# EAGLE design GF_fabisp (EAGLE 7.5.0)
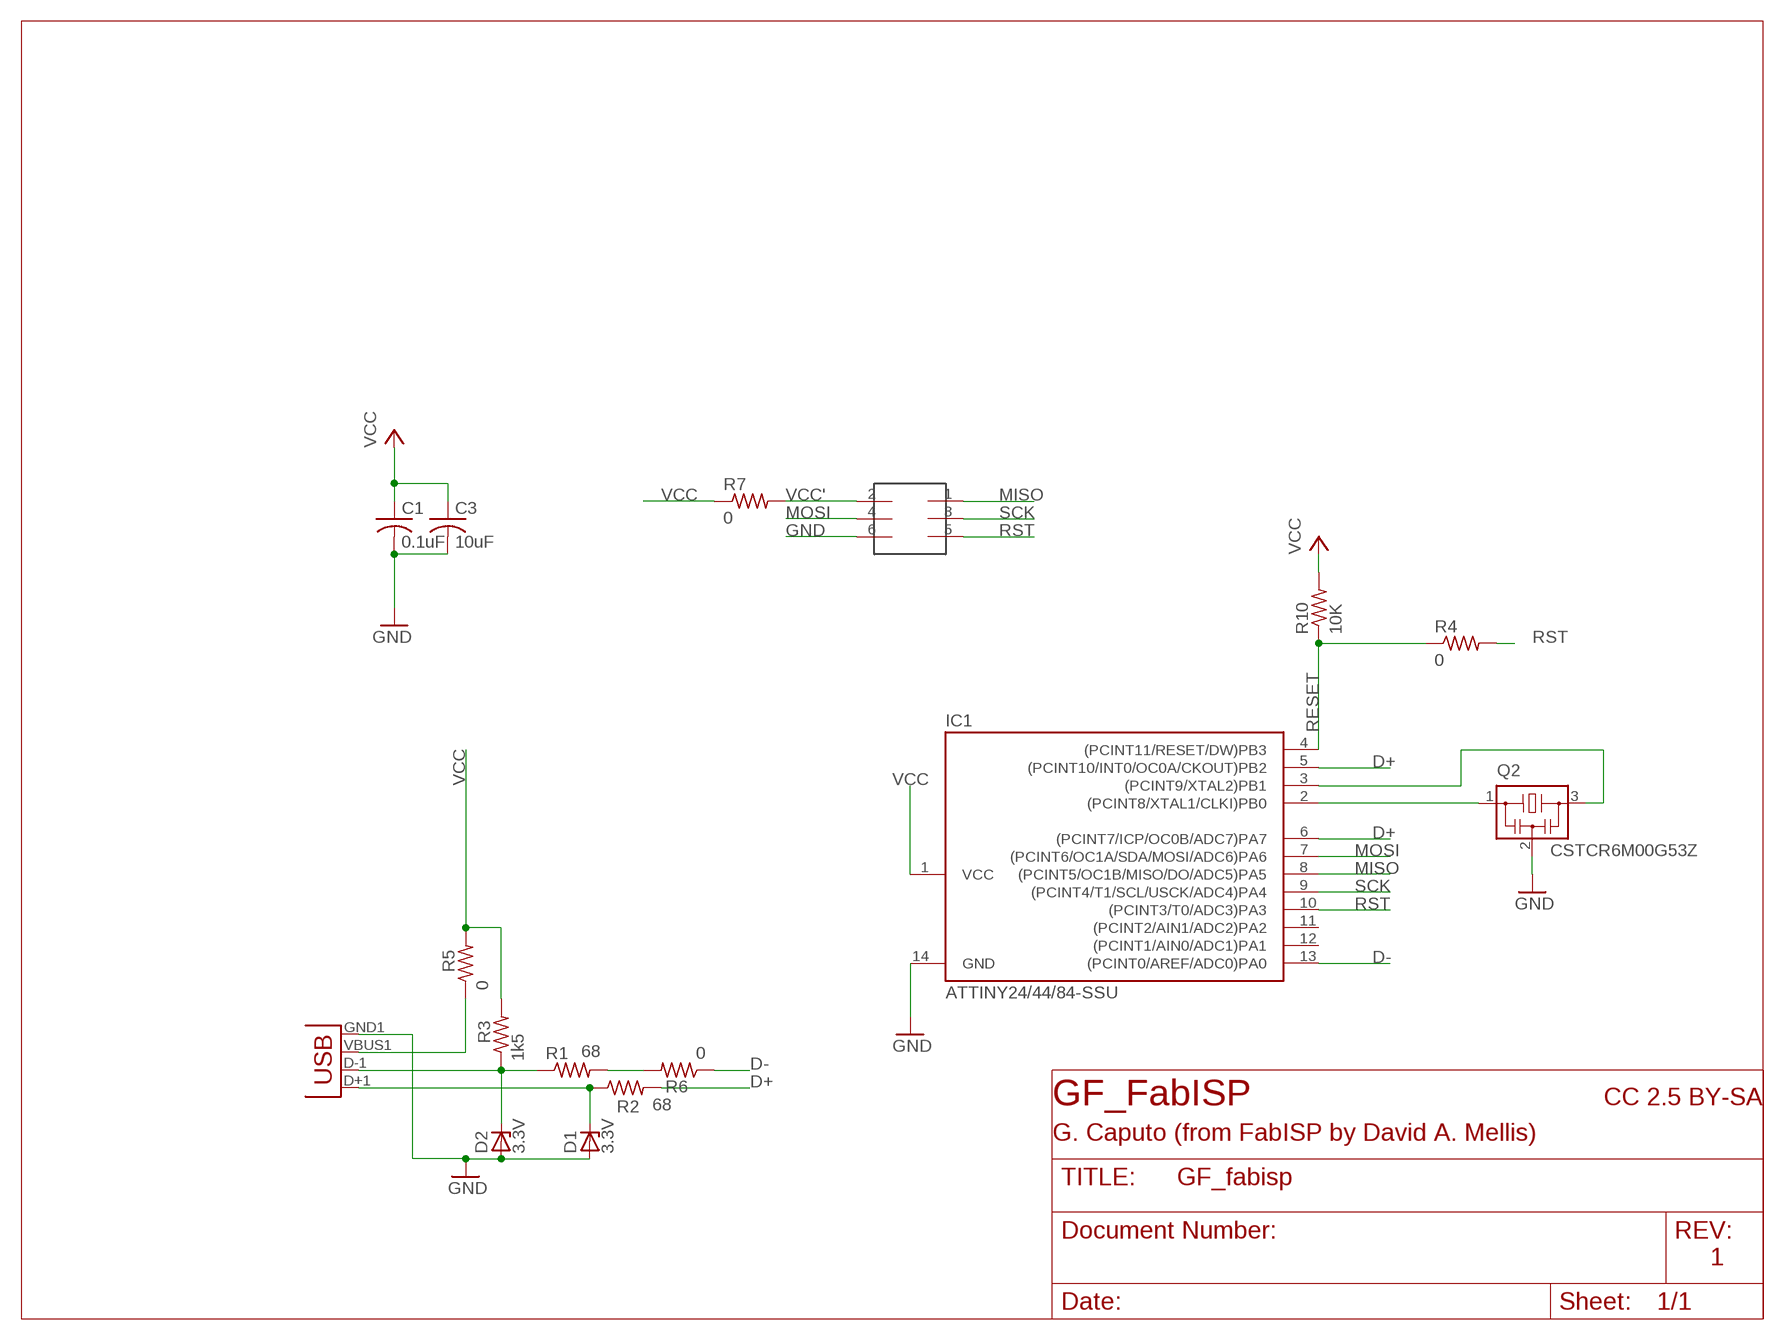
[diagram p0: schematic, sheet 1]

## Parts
C1  0.1uF  C-USC1206  [C1206]
C3  10uF  C-USC1206  [C1206]
D1  3.3V  ZENER_DIODESOD123  [SOD123]
D2  3.3V  ZENER_DIODESOD123  [SOD123]
IC1  ATTINY24/44/84-SSU  [SOIC14]
JP1  USBA-SMD-MALE  [USB-A-SMT-MALE]
Q2  CSTCR6M00G53Z  [CSTCR6M]
R1  68  R-US_R1206  [R1206]
R2  68  R-US_R1206  [R1206]
R3  1k5  R-US_R1206  [R1206]
R4  0  R-US_R1206  [R1206]
R5  0  R-US_R1206  [R1206]
R6  0  R-US_R1206  [R1206]
R7  0  R-US_R1206  [R1206]
R10  10K  R-US_R1206  [R1206]
U$1  2X3HEADER  [2X3_SMD]

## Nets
D+: IC1.5((PCINT10/INT0/OC0A/CKOUT)PB2) IC1.6((PCINT7/ICP/OC0B/ADC7)PA7) R2.2
D-: IC1.13((PCINT0/AREF/ADC0)PA0) R6.1
GND: C1.2 C3.2 D1.ANODE D2.ANODE IC1.14(GND) JP1.GND1(GND) Q2.2 U$1.6
MISO: IC1.8((PCINT5/OC1B/MISO/DO/ADC5)PA5) U$1.1
MOSI: IC1.7((PCINT6/OC1A/SDA/MOSI/ADC6)PA6) U$1.4
N$1: D2.CATHODE JP1.D-1(D-) R1.1 R3.1
N$2: D1.CATHODE JP1.D+1(D+) R2.1
N$4: IC1.2((PCINT8/XTAL1/CLKI)PB0) Q2.1
N$5: IC1.3((PCINT9/XTAL2)PB1) Q2.3
N$6: JP1.VBUS1(VBUS) R5.1
N$7: R1.2 R6.2
RESET: IC1.4((PCINT11/RESET/DW)PB3) R4.1 R10.1
RST: IC1.10((PCINT3/T0/ADC3)PA3) R4.2 U$1.5
SCK: IC1.9((PCINT4/T1/SCL/USCK/ADC4)PA4) U$1.3
VCC: C1.1 C3.1 IC1.1(VCC) R3.2 R5.2 R7.1 R10.2
VCC': R7.2 U$1.2
Unconnected: IC1.11((PCINT2/AIN1/ADC2)PA2) IC1.12((PCINT1/AIN0/ADC1)PA1)

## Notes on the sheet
- GF_FabISP | CC 2.5 BY-SA
- G. Caputo (from FabISP by David A. Mellis)
- 1

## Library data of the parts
C1 = rcl-ez:C-US: CAPACITOR, American symbol
C3 = rcl:C-US: CAPACITOR, American symbol
D1 D2 = ng:ZENER_DIODE: zener diode
IC1 = attiny24_44_84:ATTINY24/44/84
JP1 = SparkFun-Connectors:USB: USB Connectors USB-B-PTH is fully proven SKU : PRT-00139/CONN-08278 USB-miniB is fully proven SKU : PRT-00587 USB-A-PCB is untested. USB-A-H is throughly reviewed, but untested. Spark Fun Electronics SKU : PRT-00437 USB-B-SMT is throughly reviewed, but untested. Needs silkscreen touching up.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
Q2 = FablabTorino:CSTCR: Resonator Source: murata.co.jp; MPN: CSTCR6M00G53-R0; OC_FARNELL: 1170434; OC_NEWARK: 25M8759
R1-R3 R5 R6 R10 = rcl-ez:R-US_: RESISTOR, American symbol
R4 R7 = rcl:R-US_: RESISTOR, American symbol
U$1 = mellis:2X3HEADER

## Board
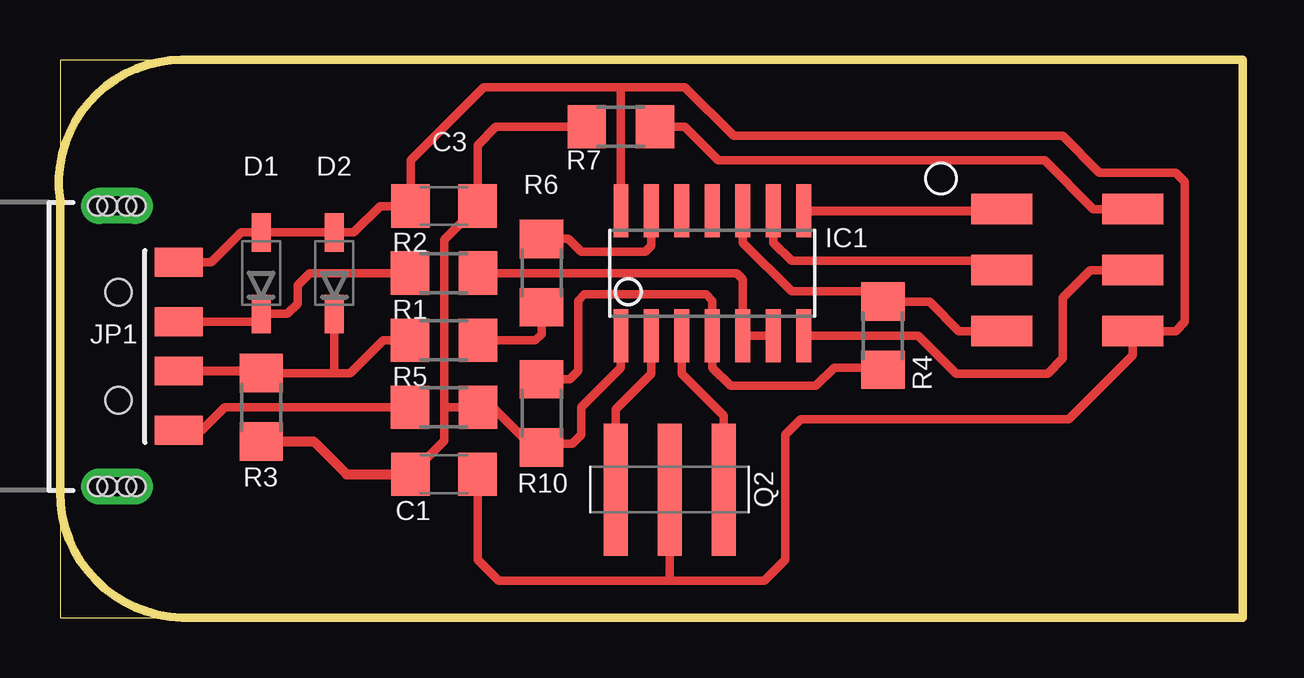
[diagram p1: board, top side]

Size 49.33 x 23.23 mm. Coordinates in mm from the lower left corner, seen from the top.
Outline: 0,0 49.33,0 49.33,23.23 0,23.23 0,0
Copper layers (1*16): Top 0.035mm / dielectric 1.5mm / Bottom 0.035mm
Design rules "default": minimum track width 10mil, minimum drill 24mil, track to track 8mil, track to pad 8mil, pad to pad 8mil, via to via 8mil, smd to smd 8mil, copper to edge 40mil, drill to drill 8mil, minimum pad ring 10mil, minimum via ring 8mil, stop-mask expansion 4mil, vias tented up to drill 0mil, thermal gap 10mil
Milling: 6 lines

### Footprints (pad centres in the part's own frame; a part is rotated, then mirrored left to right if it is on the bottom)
C1206 = smd 1.6 x 1.8: 1 -1.4,0; 2 1.4,0
SOD123 = smd 1.6 x 0.8: ANODE 1.7,0; CATHODE -1.7,0
SOIC14 = smd 0.61 x 2.21: 1 -3.81,-2.603; 2 -2.54,-2.603; 3 -1.27,-2.603; 4 0,-2.603; 5 1.27,-2.603; 6 2.54,-2.603; 7 3.81,-2.603; 8 3.81,2.603; 9 2.54,2.603; 10 1.27,2.603; 11 0,2.603; 12 -1.27,2.603; 13 -2.54,2.603; 14 -3.81,2.603
USB-A-SMT-MALE = smd 1.2 x 2: D+1 1.027,-3.67; D-1 -1.027,-3.67; GND1 3.5,-3.67; VBUS1 -3.5,-3.67 | drill 0.8 pad 1.5 long: P$1 5.85,-1.1; P$3 -5.85,-1.1 | hole 1.1: 2.25,-1.17; -2.25,-1.17 | hole 0.8: -5.85,-1.5; -5.85,-1.9; -5.85,-0.7; -5.85,-0.3; 5.85,-1.5; 5.85,-1.9; 5.85,-0.7; 5.85,-0.3
CSTCR6M = smd 1 x 5.5: 1 -2.25,0; 2 0,0; 3 2.25,0
R1206 = smd 1.6 x 1.803: 1 -1.422,0; 2 1.422,0
2X3_SMD = smd 2.54 x 1.27: 1 -2.54,2.54; 2 2.92,2.54; 3 -2.54,0; 4 2.92,0; 5 -2.54,-2.54; 6 2.92,-2.54

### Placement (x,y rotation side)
C1  16,5.97 0 top
C3  16,17.14 180 top
D1  8.38,14.35 90 top
D2  11.43,14.35 90 top
IC1  27.18,14.35 0 top
JP1  1.27,11.3 90 top
Q2  25.4,5.33 0 top
R1  16,11.56 0 top
R2  16,14.35 0 top
R3  8.38,8.76 270 top
R4  34.29,11.75 90 top
R5  16,8.76 0 top
R6  20.07,14.35 270 top
R7  23.37,20.45 0 top
R10  20.07,8.51 270 top
U$1  41.78,14.48 0 top

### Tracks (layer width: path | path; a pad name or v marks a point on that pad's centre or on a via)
D+
  Top 0.35: R2.2 28.19,14.35 28.45,14.1 IC1.5 IC1.6
D-
  Top 0.35: R6.1 21.18,15.77 21.72,15.24 24.38,15.24 24.64,15.49 IC1.13
GND
  Top 0.35: IC1.14 23.37,22.1 | C1.2 17.4,2.41 18.29,1.52 25.4,1.52 | 25.4,1.52 29.34,1.52 30.23,2.41 30.23,7.62 30.86,8.26 42.04,8.26 44.7,10.92 U$1.6 46.48,11.94 46.86,12.32 46.86,18.16 46.48,18.54 43.31,18.54 41.78,20.07 28.07,20.07 26.04,22.1 23.37,22.1 | Q2.2 25.4,1.52 | JP1.GND1 6.29,14.8 7.54,16.05 D1.ANODE D2.ANODE 12.24,16.05 13.34,17.14 C3.2 14.61,19.05 17.65,22.1 23.37,22.1
MISO
  Top 0.38: IC1.8 39.18,16.95 U$1.1
MOSI
  Top 0.35: IC1.7 35.75,11.75 37.34,10.16 41.15,10.16 41.78,10.79 41.78,13.34 42.93,14.48 U$1.4
N$1
  Top 0.35: R3.1 11.43,10.19 | 11.43,10.19 12.09,10.19 13.46,11.56 R1.1 | D2.CATHODE 11.43,10.19
  Top 0.38: JP1.D-1 8.29,10.28 R3.1
N$2
  Top 0.35: JP1.D+1 8.06,12.33 D1.CATHODE 9.48,12.65 9.91,13.08 9.91,13.84 10.41,14.35 R2.1
N$4
  Top 0.35: IC1.2 24.64,10.16 23.15,8.67 Q2.1
N$5
  Top 0.35: IC1.3 25.91,10.16 27.65,8.42 Q2.3
N$6
  Top 0.35: JP1.VBUS1 5.9,7.8 6.86,8.76 R5.1
N$7
  Top 0.35: R1.2 19.81,11.56 20.07,11.81 R6.2
RESET
  Top 0.35: R10.1 21.23,9.93 21.59,10.29 21.59,13.21 21.84,13.46 26.92,13.46 27.18,13.21 IC1.4 27.18,10.41 27.94,9.65 31.5,9.65 32.26,10.41 34.27,10.41 R4.1
RST
  Top 0.35: IC1.10 28.45,15.62 30.48,13.59 33.93,13.59 R4.2 | U$1.5 37.45,11.94 36.23,13.16 34.3,13.16
  Top 0.38: 34.3,13.16 R4.2
SCK
  Top 0.35: IC1.9 29.72,15.62 30.48,14.86 38.86,14.86 U$1.3
VCC
  Top 0.35: 19.91,7.24 19.56,7.24 18.03,8.76 R5.2 16.13,8.76 16,8.89 | 19.91,7.24 R10.2 | 19.91,7.24 21.34,7.24 21.72,7.62 21.72,8.76 23.37,10.41 IC1.1 | R7.1 18.16,20.45 17.4,19.69 C3.1 16,15.74 16,8.89 | C1.1 16,7.37 16,8.89
  Top 0.406: R3.2 10.57,7.34 11.94,5.97 C1.1
VCC'
  Top 0.35: U$1.2 43.05,17.02 41.02,19.05 27.43,19.05 26.04,20.45 R7.2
